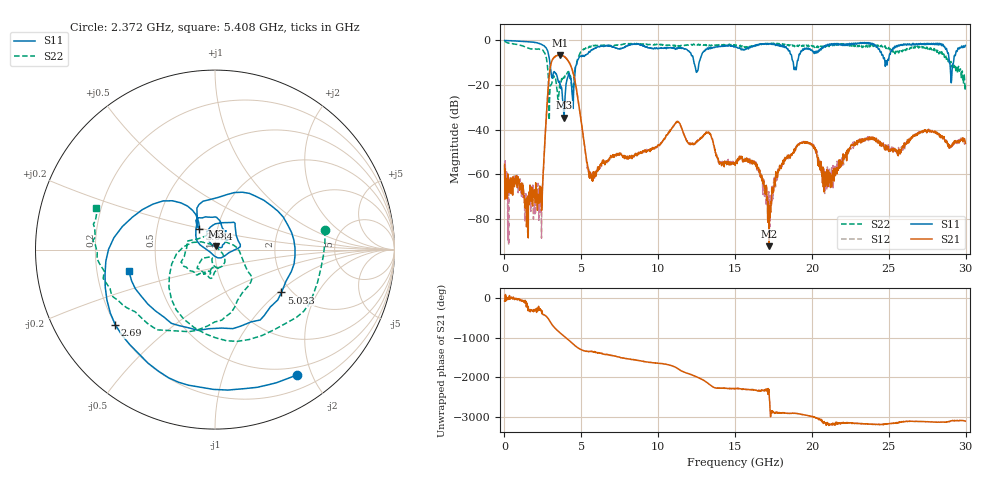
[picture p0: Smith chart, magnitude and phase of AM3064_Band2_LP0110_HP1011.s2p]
# Hz S DB R 50.0
!freq dBS11 angS11 dBS21 angS21 dBS12 angS12 dBS22 angS22
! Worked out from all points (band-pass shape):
!   1600 points, 10 MHz to 29.98 GHz, reference 50 ohm
!   highest |S21| = -6.49 dB at 3.59 GHz (marker M1); lowest = -92.1 dB at 17.22 GHz (marker M2)
!   |S21| within 3 dB of the highest: 3.064 GHz to 4.179 GHz (1.115 GHz wide, 30.8 % of centre)
!   lowest |S11| = -34.6 dB at 3.871 GHz (marker M3), VSWR 1.04, Z = 50.5 + j1.8 ohm
!   |S11| at or under -10 dB: 2.956 GHz to 4.716 GHz (1.76 GHz wide, 45.9 % of centre); 12.33 GHz to 12.66 GHz (327.3 MHz wide, 2.62 % of centre); 28.95 GHz to 29.2 GHz (255.8 MHz wide, 0.88 % of centre)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
!   |S22| runs from -35.7 to -0.3 dB; largest |S21 - S12| = 0.015
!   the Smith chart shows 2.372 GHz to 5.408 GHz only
!   S11 on the Smith chart (normalised r, x): 2.372 GHz: 0.39, -1.78; 2.69 GHz: 0.20, -0.32; 3.084 GHz: 0.82, +0.20; 5.033 GHz: 1.78, -1.05; 5.408 GHz: 0.34, -0.11
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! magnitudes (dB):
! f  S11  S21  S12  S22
! 10 MHz  0.0  -55.4  -55.8  -0.3
! 2.372 GHz  -1.6  -65.7  -69.6  -4.1
! 2.69 GHz  -3.1  -37.8  -37.7  -7.0
! 3.084 GHz  -16.7  -9.3  -9.1  -18.9
! 3.59 GHz  -18.4  -6.5  -6.6  -19.8
! 3.871 GHz  -34.6  -7.1  -7.1  -16.6
! 5.015 GHz  -7.3  -37.2  -37.1  -5.1
! 5.033 GHz  -7.1  -38.2  -38.1  -5.0
! 5.408 GHz  -6.1  -55.9  -56.3  -3.1
! 10 GHz  -3.6  -46.6  -46.8  -1.9
! 11.27 GHz  -3.6  -36.3  -36.2  -2.5
! 12.49 GHz  -14.3  -45.2  -45.8  -1.9
! 15 GHz  -2.6  -55.9  -54.8  -2.1
! 16.39 GHz  -2.1  -56.0  -55.8  -2.2
! 17.22 GHz  -1.5  -92.1  -81.1  -1.5
! 18.17 GHz  -2.6  -53.6  -54.4  -2.1
! 19.99 GHz  -4.3  -46.8  -46.9  -2.3
! 20.89 GHz  -2.2  -65.3  -61.1  -2.9
! 23.12 GHz  -1.4  -44.2  -44.6  -3.0
! 25 GHz  -8.3  -49.7  -48.9  -3.2
! 29.08 GHz  -17.8  -47.0  -47.2  -10.8
! 29.98 GHz  -2.3  -46.0  -46.6  -20.2
